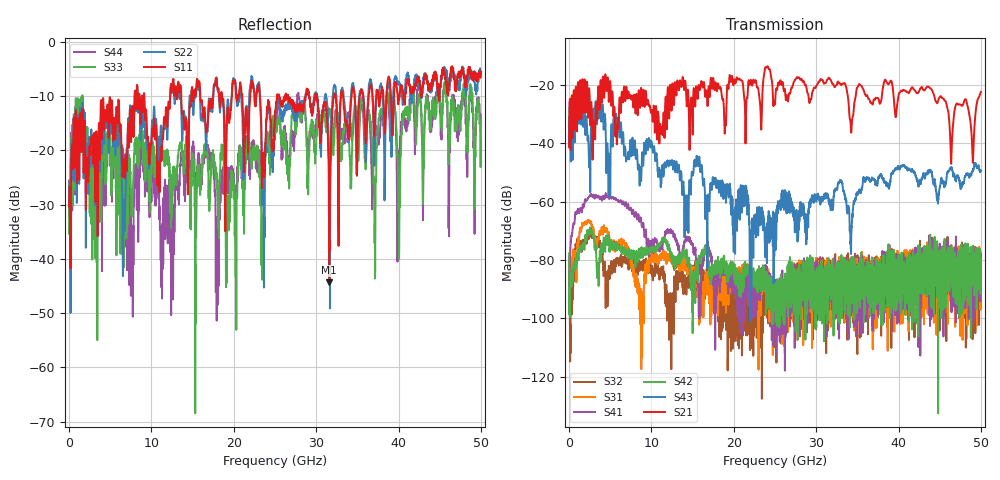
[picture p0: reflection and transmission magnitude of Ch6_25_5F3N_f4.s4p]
!Agilent Technologies,N5247A,US51170199,A.09.90.13
!Agilent N5247A: A.09.90.13
!Date: Wednesday, December 16, 2015 09:46:38
!Correction: S11(Full 4 Port(1,2,3,4))
!S12(Full 4 Port(1,2,3,4))
!S13(Full 4 Port(1,2,3,4))
!S14(Full 4 Port(1,2,3,4))
!S21(Full 4 Port(1,2,3,4))
!S22(Full 4 Port(1,2,3,4))
!S23(Full 4 Port(1,2,3,4))
!S24(Full 4 Port(1,2,3,4))
!S31(Full 4 Port(1,2,3,4))
!S32(Full 4 Port(1,2,3,4))
!S33(Full 4 Port(1,2,3,4))
!S34(Full 4 Port(1,2,3,4))
!S41(Full 4 Port(1,2,3,4))
!S42(Full 4 Port(1,2,3,4))
!S43(Full 4 Port(1,2,3,4))
!S44(Full 4 Port(1,2,3,4))
!S4P File: Measurements: <S11,S12,S13,S14>,
!<S21,S22,S23,S24>,
!<S31,S32,S33,S34>,
!<S41,S42,S43,S44>:
# Hz S  dB  R 50
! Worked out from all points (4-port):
!   3201 points, 10 MHz to 50 GHz, reference 50 ohm
!   strongest paths, dB at 10 MHz, 12.51 GHz, 25 GHz, 37.5 GHz, 50 GHz:
!     S21: -41.4, -21.5, -26.7, -24.6, -22.5
!     S43: -40.9, -46.2, -74.6, -52.7, -49.3
!     S42: -77.7, -81.2, -91.4, -88.7, -85.7
!     S41: -88.7, -70.8, -98.9, -84.3, -85.3
!     S31: -84.6, -80.2, -94.6, -88.4, -85.6
!     S32: -79.1, -92.9, -96.3, -85.9, -83.0
!   lowest |S11| = -44.3 dB at 31.58 GHz (marker M1), VSWR 1.01, Z = 49.4 + j0.0648 ohm
!   |S11| at or under -10 dB: start of sweep to 7.958 GHz; 9.143 GHz to 12.29 GHz (3.145 GHz wide, 29.4 % of centre); 26.6 GHz to 28.71 GHz (2.111 GHz wide, 7.63 % of centre)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
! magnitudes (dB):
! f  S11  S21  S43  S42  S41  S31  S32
! 10 MHz  -30.4  -41.4  -40.9  -77.7  -88.7  -84.6  -79.1
! 2.759 GHz  -18.8  -28.4  -33.3  -70.3  -57.8  -68.1  -72.0
! 22.15 GHz  -7.1  -19.2  -81.3  -86.9  -98.4  -87.5  -91.1
! 23.63 GHz  -23.4  -17.5  -69.5  -88.6  -83.0  -86.3  -95.4
! 31.58 GHz  -44.3  -17.6  -59.3  -91.6  -96.9  -93.4  -91.9
! 46.41 GHz  -5.1  -46.2  -48.9  -83.3  -84.4  -81.8  -97.5
! 50 GHz  -5.6  -22.5  -49.3  -85.7  -85.3  -85.6  -83.0
